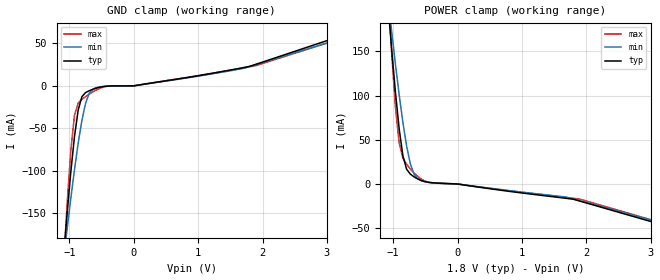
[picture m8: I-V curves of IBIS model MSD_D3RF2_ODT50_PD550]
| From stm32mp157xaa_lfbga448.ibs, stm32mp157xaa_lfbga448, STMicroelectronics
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[Model] MSD_D3RF2_ODT50_PD550
Model_type   Input
C_comp 2.311pF   2.272pF   2.340pF
Vinh = 1.150V
Vinl = 650.000mV
[Temperature Range]   25.000   125.000   -40.000
[Voltage Range]   1.800V   1.700V   1.900V
[GND Clamp Reference]   0.00V   0.00V   0.00V
[POWER Clamp Reference]   1.800V   1.700V   1.900V
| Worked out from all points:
|   GND clamp passes 1 mA (typ) near -0.48 V on its own axis
|   POWER clamp passes 1 mA (typ) near -0.31 V on its own axis
[GND Clamp]
-1.785V   -919.9mA   -680.4mA   -1.29A
-1.094V   -205.1mA   -206.4mA   -215.3mA
-1.036V   -151.4mA   -169.2mA   -139.9mA
-978.8mV  -102.1mA   -133.2mA   -76.95mA
-921.2mV  -59.88mA   -99mA      -34.81mA
-863.6mV  -28.55mA   -67.7mA    -20.3mA
-806.1mV  -12.85mA   -40.83mA   -15.95mA
-748.5mV  -7.942mA   -20.47mA   -12.71mA
-690.9mV  -5.718mA   -8.568mA   -9.738mA
-575.8mV  -2.61mA    -2.002mA   -4.6mA
1.785V    22.71mA    22.43mA    22.19mA
3.57V     67.67mA    63.59mA    64.14mA
[Power Clamp]
-1.77V    921.4mA    689.4mA    1.288A
-1.079V   202.9mA    209.2mA    217.9mA
-1.021V   150.6mA    171.6mA    146.6mA
-963.6mV  103.1mA    135.1mA    86.31mA
-906.1mV  62.17mA    100.7mA    46.02mA
-848.5mV  31.8mA     69.4mA     29.28mA
-790.9mV  16.69mA    42.82mA    22.34mA
-733.3mV  11.19mA    22.93mA    17.02mA
-618.2mV  5.714mA    5.783mA    8.515mA
-387.9mV  1.368mA    1.275mA    1.181mA
1.8V      -17.31mA   -16.98mA   -16.29mA
3.585V    -54.7mA    -52.23mA   -52.76mA
